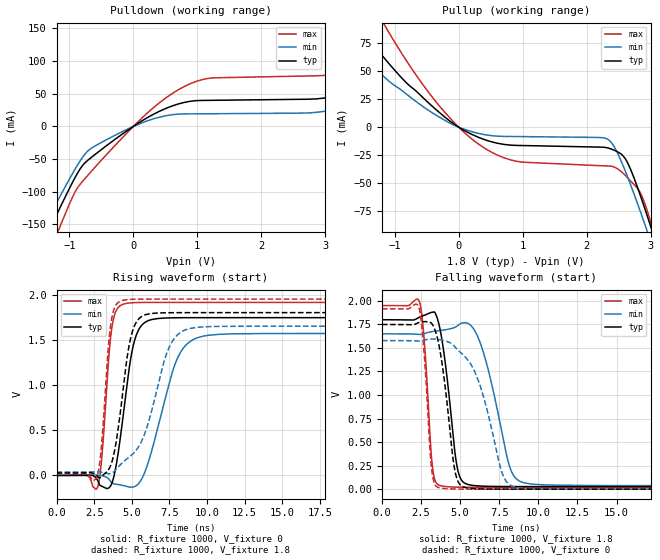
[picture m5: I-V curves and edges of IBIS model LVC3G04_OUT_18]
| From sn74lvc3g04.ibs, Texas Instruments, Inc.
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[Model]   LVC3G04_OUT_18
Model_type  Output
Vref =   0
Rref =   1000
Cref =   30p
Vmeas =   0.9
| variable   typ   min   max
C_comp   9.93pF   6.40pF   16.19pF
| C_pullup   9.15pF   6.40pF   10.36pF
| C_pulldown   10.70pF   6.76pF   16.19pF
[Temperature Range]   40   100   -40
| Ambient temperature   25   85   -40
[Voltage range]   1.8   1.65   1.95
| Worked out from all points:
|   slope of the pulldown table from 0 to 0.27 V, typ, clamps not added: 16.6 ohm
|   slope of the pullup table from 0 to 0.27 V, typ, clamps not added: 33.1 ohm
|   rising waveform, R_fixture 1000, V_fixture 0: 20-80 % time 864ps typ, 1.55ns min, 502ps max; typ from 0 V to 1.74 V
|   falling waveform, R_fixture 1000, V_fixture 1.8: 20-80 % time 711ps typ, 1.27ns min, 427ps max; typ from 1.8 V to 0.027 V
|   rising waveform, R_fixture 1000, V_fixture 1.8: 20-80 % time 861ps typ, 1.68ns min, 500ps max; typ from 0.027 V to 1.8 V
|   falling waveform, R_fixture 1000, V_fixture 0: 20-80 % time 741ps typ, 1.55ns min, 430ps max; typ from 1.75 V to 0 V
[Pulldown]
| LVC3G04_OUT_18
|   Voltage   I(typ)   I(min)   I(max)
-5V       -921.3mA   -834.5mA   -1.063A
-1.445V   -186.3mA   -162.4mA   -225.4mA
-1.25V    -145.7mA   -126mA     -178.1mA
-685mV    -49.64mA   -35.35mA   -71.84mA
610mV     31.45mA    17.97mA    50.48mA
1.215V    39.94mA    19.45mA    74.07mA
3.215V    47.58mA    27.04mA    81.89mA
3.75V     64.33mA    35.96mA    102.6mA
4.19V     79.14mA    21.53mA    128.3mA
4.615V    44.44mA    21.76mA    152.7mA
5.01V     44.71mA    21.99mA    83.17mA
10V       49.72mA    24.78mA    91.33mA
[Pullup]
| LVC3G04_OUT_18
|   Voltage   I(typ)   I(min)   I(max)
-5V       401.9mA    301.7mA    569.7mA
-1.995V   124.3mA    92.87mA    180.5mA
-1.525V   87.6mA     64.51mA    128.6mA
-1.245V   67.41mA    49.06mA    99.76mA
-215mV    8.959mA    6.079mA    13.21mA
460mV     -12.21mA   -7.201mA   -20.69mA
1.005V    -16.45mA   -8.461mA   -31.35mA
2.32V     -18.45mA   -10.52mA   -34.74mA
2.62V     -29.72mA   -41.55mA   -44.14mA
2.935V    -77.24mA   -91.1mA    -72.7mA
3.07V     -101mA     -113.7mA   -97.52mA
10V       -1.501A    -1.413A    -1.659A
[Ramp]
| LVC3G04_OUT_18
| variable   typ   min   max
dV/dt_r   1.13/9.33E-10   1.02/1.66E-09   1.24/5.43E-10
dV/dt_f   1.11/7.58E-10   1.04/1.40E-09   1.20/4.50E-10
R_load = 1000
[Rising Waveform]
| LVC3G04_OUT_18
R_fixture =   1000
C_fixture =   0
L_fixture =   0
V_fixture =   0
V_fixture_min = 0
V_fixture_max = 0
|   Time   V(typ)   V(min)   V(max)
0s        112.7pV    7.745nV    2.81nV
2.735ns   -55.57mV   3.176mV    -127.7mV
3.01ns    -119.5mV   -2.471mV   199.4mV
3.64ns    -101.4mV   -74.9mV    1.585V
4.335ns   534.8mV    -108.1mV   1.887V
4.975ns   1.333V     -131mV     1.909V
5.54ns    1.633V     -72.47mV   1.912V
7.9ns     1.743V     1.239V     1.913V
9.135ns   1.744V     1.506V     1.913V
24.99ns   1.744V     1.569V     1.913V
[Falling Waveform]
| LVC3G04_OUT_18
R_fixture =   1000
C_fixture =   0
L_fixture =   0
V_fixture =   1.8
V_fixture_min = 1.65
V_fixture_max = 1.95
|   Time   V(typ)   V(min)   V(max)
0s        1.8V       1.65V      1.95V
2.41ns    1.827V     1.643V     1.988V
2.71ns    1.847V     1.652V     1.578V
3.21ns    1.879V     1.673V     274.2mV
3.625ns   1.769V     1.683V     44.61mV
4.77ns    275.6mV    1.727V     21.67mV
5.33ns    60.67mV    1.769V     20.32mV
6.36ns    32.95mV    1.521V     19.67mV
8.805ns   27.4mV     85.21mV    19.52mV
24.99ns   26.98mV    37.55mV    19.51mV
[Rising Waveform]
| LVC3G04_OUT_18
R_fixture =   1000
C_fixture =   0
L_fixture =   0
V_fixture =   1.8
V_fixture_min = 1.65
V_fixture_max = 1.95
|   Time   V(typ)   V(min)   V(max)
0s        26.95mV    37.49mV    19.5mV
2.69ns    -5.295mV   40.15mV    -15.39mV
2.98ns    -14.74mV   35.86mV    312.2mV
3.59ns    106.5mV    19.68mV    1.651V
4.225ns   675.7mV    114.9mV    1.925V
4.8ns     1.414V     199.8mV    1.946V
5.32ns    1.699V     284.4mV    1.949V
7.4ns     1.799V     1.381V     1.95V
8.49ns    1.8V       1.604V     1.95V
24.99ns   1.8V       1.65V      1.95V
[Falling Waveform]
| LVC3G04_OUT_18
R_fixture =   1000
C_fixture =   0
L_fixture =   0
V_fixture =   0
V_fixture_min = 0
V_fixture_max = 0
|   Time   V(typ)   V(min)   V(max)
0s        1.749V     1.578V     1.916V
2.39ns    1.772V     1.573V     1.919V
2.685ns   1.78V      1.581V     1.486V
3.165ns   1.764V     1.595V     241.4mV
3.585ns   1.581V     1.591V     19.52mV
4.635ns   227.4mV    1.52V      1.79mV
5.195ns   24.59mV    1.427V     633.3uV
6.14ns    3.851mV    1.166V     138.9uV
8.33ns    286.2uV    31.73mV    22.46uV
24.99ns   22.05uV    44.1uV     12.65uV
